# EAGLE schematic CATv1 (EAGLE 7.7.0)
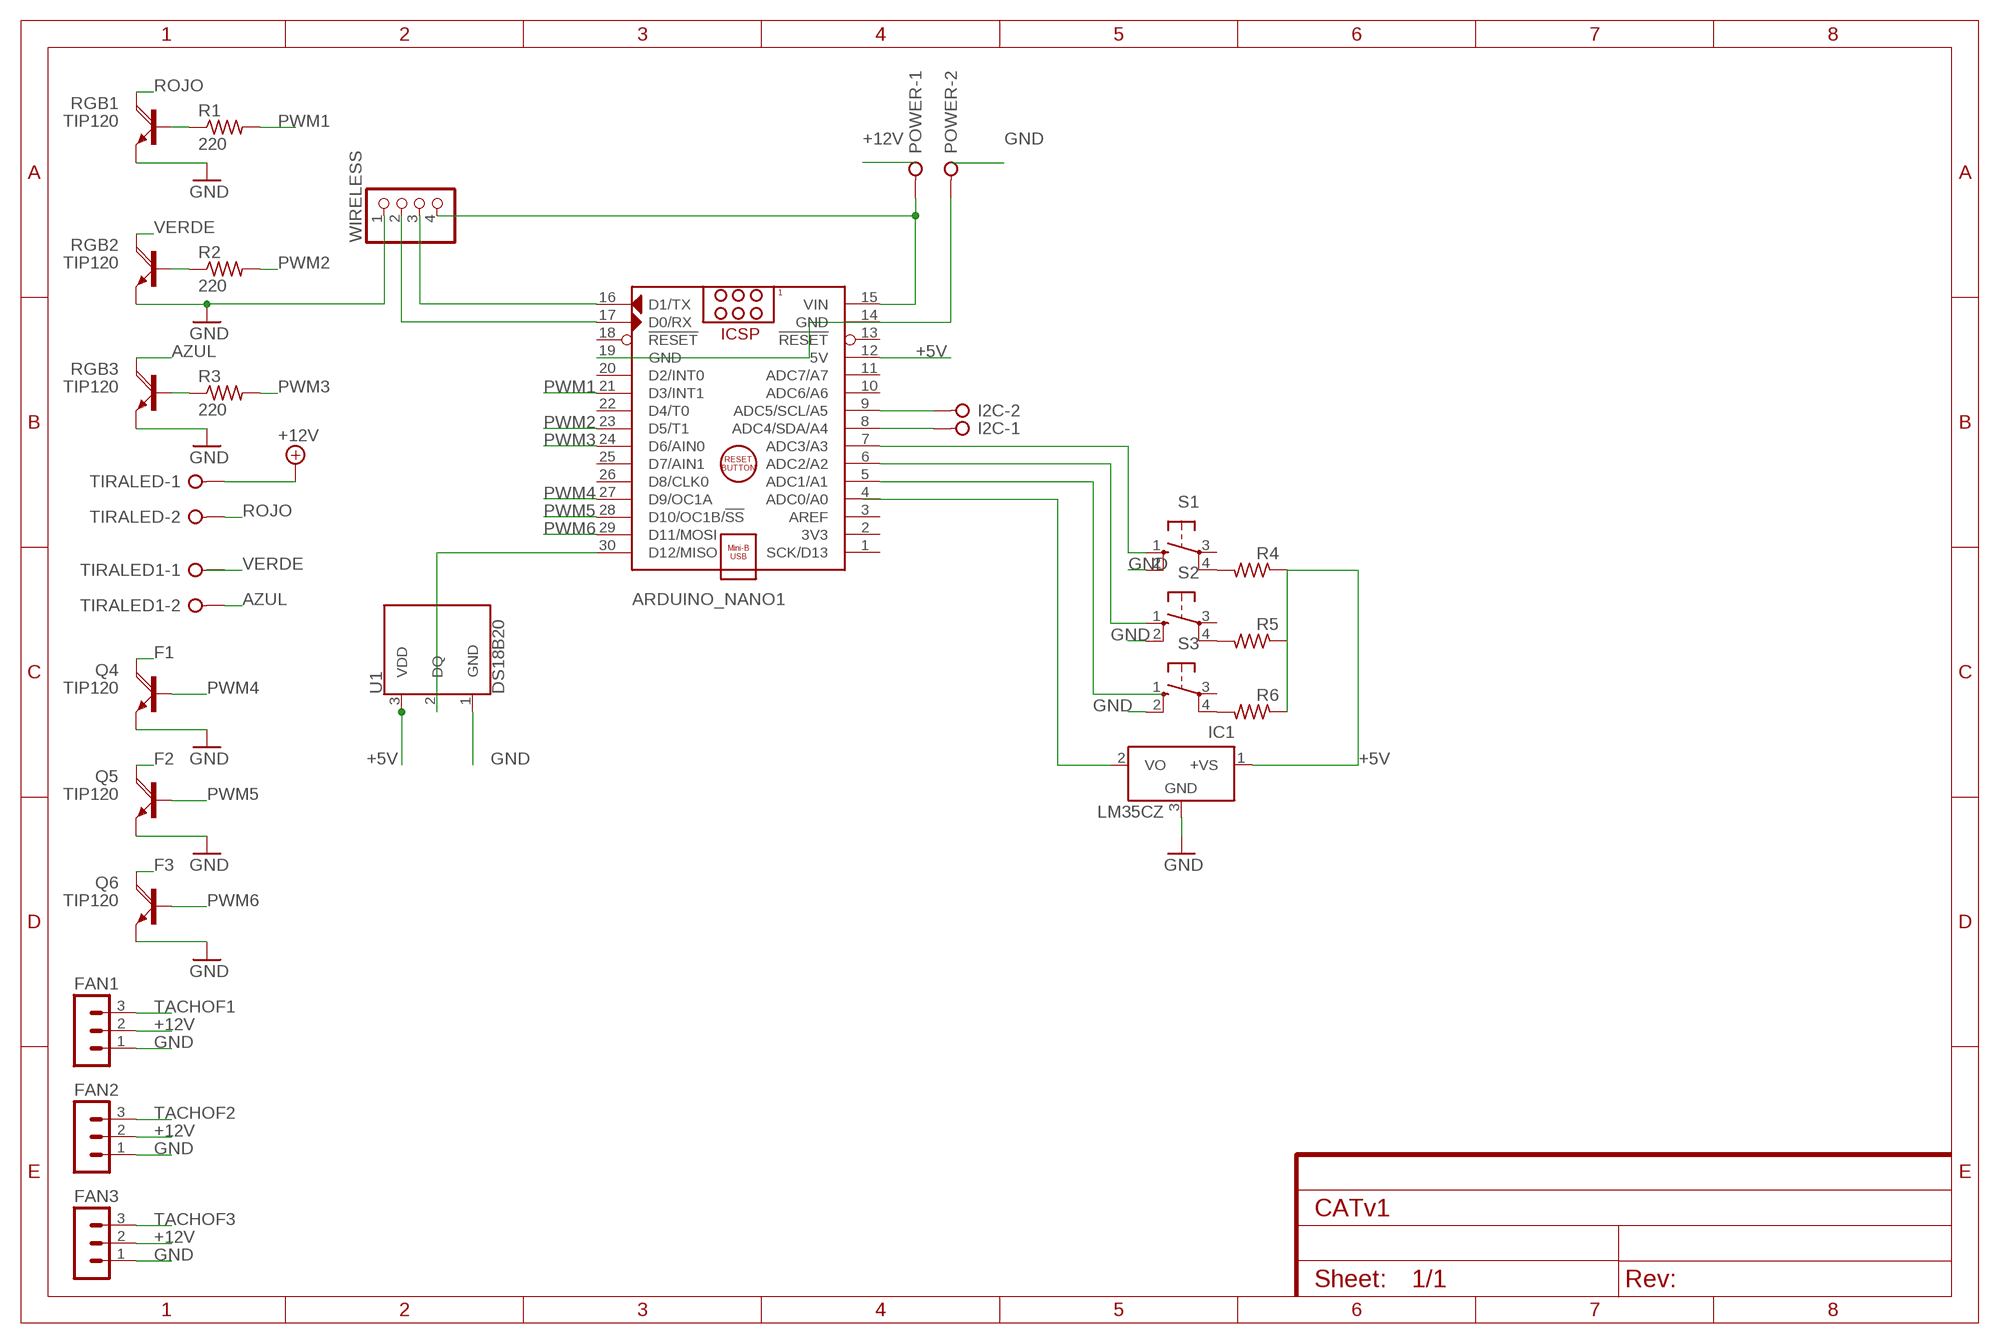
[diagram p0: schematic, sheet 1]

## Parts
ARDUINO_NANO1  ARDUINO_NANO  [ARDUINO_NANO]
FAN1  MA03-1  [MA03-1]
FAN2  MA03-1  [MA03-1]
FAN3  MA03-1  [MA03-1]
I2C  W237-02P  [W237-132]
IC1  LM35CZ  [TO92]
POWER  W237-02P  [W237-132]
Q4  TIP120  [TO220AH]
Q5  TIP120  [TO220AH]
Q6  TIP120  [TO220AH]
R1  220  R-US_0207/10  [0207/10]
R2  220  R-US_0207/10  [0207/10]
R3  220  R-US_0207/10  [0207/10]
R4  R-US_0207/10  [0207/10]
R5  R-US_0207/10  [0207/10]
R6  R-US_0207/10  [0207/10]
RGB1  TIP120  [TO220AH]
RGB2  TIP120  [TO220AH]
RGB3  TIP120  [TO220AH]
S1  10-XX  [B3F-10XX]
S2  10-XX  [B3F-10XX]
S3  10-XX  [B3F-10XX]
TIRALED  W237-02P  [W237-132]
TIRALED1  W237-02P  [W237-132]
U1  DS18B20  [TO-92-AMMO]
WIRELESS  PINHD-1X4  [1X04]

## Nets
+5V: ARDUINO_NANO1.12(5V) IC1.1(+VS) R4.1 R5.1 R6.1 U1.3(VDD)
+12V: FAN1.2 FAN2.2 FAN3.2 TIRALED.1
AZUL: RGB3.C TIRALED1.2
F1: Q4.C
F2: Q5.C
F3: Q6.C
GND: ARDUINO_NANO1.14(GND) ARDUINO_NANO1.19(GND) FAN1.1 FAN2.1 FAN3.1 IC1.3(GND) POWER.2 Q4.E Q5.E Q6.E RGB1.E RGB2.E RGB3.E S1.2(S1) S2.2(S1) S3.2(S1) U1.1(GND) WIRELESS.1
N$1: ARDUINO_NANO1.16(D1/TX) WIRELESS.3
N$2: ARDUINO_NANO1.17(D0/RX) WIRELESS.2
N$3: ARDUINO_NANO1.15(VIN) POWER.1 WIRELESS.4
N$4: R1.1 RGB1.B
N$5: R2.1 RGB2.B
N$6: R3.1 RGB3.B
N$7: ARDUINO_NANO1.30(D12/MISO) U1.2(DQ)
N$8: ARDUINO_NANO1.9(ADC5/SCL/A5) I2C.2
N$9: ARDUINO_NANO1.8(ADC4/SDA/A4) I2C.1
N$10: IC1.2(VO)
N$11: ARDUINO_NANO1.7(ADC3/A3) S1.1(S)
N$12: R4.2 S1.4(P1)
N$13: R5.2 S2.4(P1)
N$14: R6.2 S3.4(P1)
N$15: ARDUINO_NANO1.6(ADC2/A2) S2.1(S)
N$16: ARDUINO_NANO1.5(ADC1/A1)
PWM1: ARDUINO_NANO1.21(D3/INT1) R1.2
PWM2: ARDUINO_NANO1.23(D5/T1) R2.2
PWM3: ARDUINO_NANO1.24(D6/AIN0) R3.2
PWM4: ARDUINO_NANO1.27(D9/OC1A) Q4.B
PWM5: ARDUINO_NANO1.28(D10/OC1B/!SS) Q5.B
PWM6: ARDUINO_NANO1.29(D11/MOSI) Q6.B
ROJO: RGB1.C TIRALED.2
TACHOF1: FAN1.3
TACHOF2: FAN2.3
TACHOF3: FAN3.3
VERDE: RGB2.C
Unconnected: ARDUINO_NANO1.1(SCK/D13) ARDUINO_NANO1.2(3V3) ARDUINO_NANO1.3(AREF) ARDUINO_NANO1.4(ADC0/A0) ARDUINO_NANO1.10(ADC6/A6) ARDUINO_NANO1.11(ADC7/A7) ARDUINO_NANO1.13(!RESET) ARDUINO_NANO1.18(!RESET) ARDUINO_NANO1.20(D2/INT0) ARDUINO_NANO1.22(D4/T0) ARDUINO_NANO1.25(D7/AIN1) ARDUINO_NANO1.26(D8/CLK0) S1.3(P) S2.3(P) S3.1(S) S3.3(P) TIRALED1.1

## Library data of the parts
ARDUINO_NANO1 = ArduinoNanoV30:ARDUINO_NANO: Arduino Nano V3.0 Module Overview: The Arduino Nano is a small, complete, and breadboard-friendly board based on the ATmega328 (Arduino Nano 3.x) or ATmega168 (Arduino Nano 2.x). It has more or less the same functionality of the Arduino Duemilanove, but in a different package. It lacks only a DC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
FAN1-FAN3 = con-lstb:MA03-1: PIN HEADER; OC_FARNELL: unknown; OC_NEWARK: unknown
I2C POWER TIRALED TIRALED1 = con-wago-508:W237-02P: WAGO SREW CLAMP; OC_FARNELL: unknown; OC_NEWARK: unknown
IC1 = lm35:LM35: Single-Supply Centigrade Temperature Sensor Vout = (10mV/°C x Temp °C) +5mmmV Source: http://www.national.com/ds/LM/LM35.pdf
Q4-Q6 RGB1-RGB3 = transistor-power:TIP120: NPN DARLINGTON TRANSISTOR
R1-R3 = adafruit:R-US_: RESISTOR, American symbol
R4-R6 = rcl:R-US_: RESISTOR, American symbol
S1-S3 = switch-omron:10-XX: OMRON SWITCH; MPN: B3F-1000; OC_FARNELL: 176432; OC_NEWARK: 36M3542
U1 = SparkFun-Sensors:DS18B20: Dallas/Maxim DS18B20 1-Wire Temperature Sensor The DS18B20 reports degrees C with 9 to 12-bit precision, -55C to 125C (+/-0.5C). Each sensor has a unique 64-Bit Serial number etched into it - allows for a huge number of sensors to be used on one data bus. Datasheet SparkFun Products One Wire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; STORE_ID: SEN-00245
WIRELESS = pinhead:PINHD-1X4: PIN HEADER

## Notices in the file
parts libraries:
SparkFun-Sensors: Licensing: Creative Commons ShareAlike 4.0 International - https://creativecommons.org/licenses/by-sa/4.0
